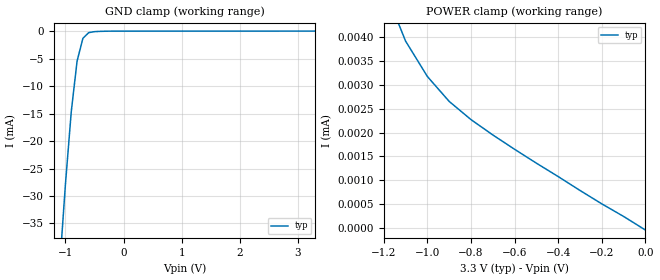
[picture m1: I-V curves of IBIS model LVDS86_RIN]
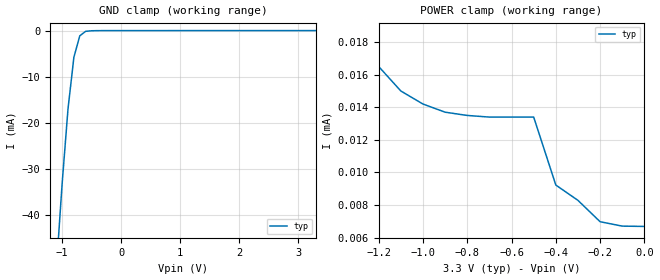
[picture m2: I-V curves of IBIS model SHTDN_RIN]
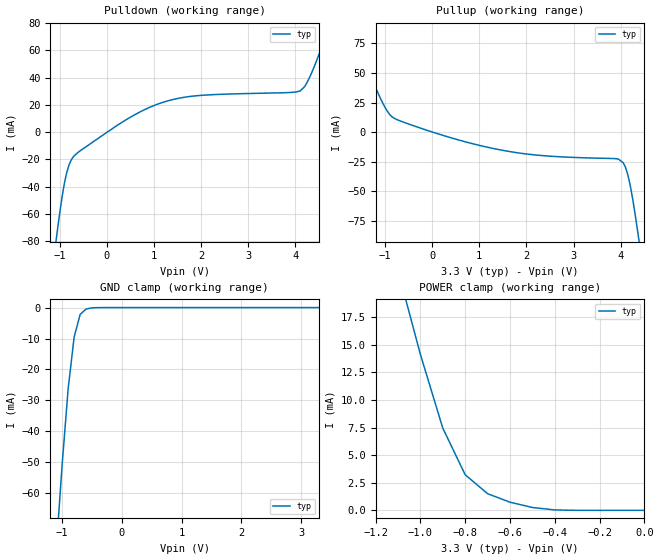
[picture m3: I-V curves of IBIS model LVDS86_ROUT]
|   Texas Instruments Incorporated
|   Data Transmissions Products
|   IBIS Model for SN75LVDS86
|   48DGG Package
[IBIS Ver]   2.1
[Comment char]   |_char
[File name]   75lvds86.ibs
[File Rev]   2.0
[Date]   21Feb97
[Source]   File originated at Texas Instruments Incorporated.
   Data Transmission Products Group. All data based on
   Bench Measurements.
[Notes]   File created by Thomas Fisher
[Disclaimer]
(C) Copyright Texas Instruments Incorporated 1997
   All rights reserved
  Texas Instruments Incorporated hereby grants the user of this IBIS
model a non-exclusive, nontransferable license to use this IBIS model
under the following terms.  Before using this IBIS model, the user
should read this license.  If the user does not accept these terms,
the IBIS model should be returned to Texas Instruments within 30 days.
  The user is granted this license only to use the IBIS model and
is not granted rights to sell, load, rent, lease or license the IBIS
model in whole or in part, or in modified form to anyone other than
user.  User may modify the IBIS model to suit its specific applications
but rights to derivative works and such modifications shall belong to
Texas Instruments.
  This IBIS model is provided on an "AS IS" basis and Texas Instruments
makes absolutely no warranty with respect to the information contained
herein.  TEXAS INSTRUMENTS DISCLAIMS AND CUSTOMER WAIVES ALL WARRANTIES,
EXPRESS OR IMPLIED, INCLUDING WARRANTIES OF MERCHANTABILITY OR FITNESS
FOR A PARTICULAR PURPOSE. The entire risk as to quality and performance
is with the Customer. ACCORDINGLY, IN NO EVENT SHALL THE COMPANY BE LIABLE
FOR ANY DAMAGES, WHETHER IN CONTRACT OR TORT,INCLUDING ANY LOST PROFITS
OR OTHER INCIDENTAL, CONSEQUENTIAL, EXEMPLARY, OR PUNITIVE DAMAGES ARISING
OUT OF THE USE OR APPLICATION OF THE IBIS model provided in this package.
Further, Texas Instruments reserves the right to discontinue or make changes
without notice to any product herein to improve reliability, function, or
design. Texas Instruments does not convey any license under patent rights
or any other intellectual property rights, including those of third parties.
Contact Texas Instruments at ATTN:DATA TRANSMISSIONS
Thomas Fisher  8505 Forest Lane, M/S 8710, Dallas, TX 75243-4136
IBIS Open Forum disclaims all warranties. See DISCLAIM.TXT
in vhdl.org:/pub/IBIS/models for the full disclaimer.
[Copyright]   Copyright 1997, Texas Instruments, All Rights Reserved
[Component]   SN75LVDS86DGG
[Manufacturer]  Texas Instruments Incorporated
[Package]
|   typ   min   max
R_pkg   0.036   0.022   0.041
L_pkg   2.128nH   2.045nH   2.336nH
C_pkg   0.357pF   0.310pF   0.394pF
[Pin]  signal_name   model_name   R_pin   L_pin   C_pin
1   D17   LVDS86_ROUT   0.041   2.221n   0.310p
2   D18   LVDS86_ROUT   0.041   2.297n   0.394p
3   GND   GND   0.022   2.336n   0.380p
4   D19   LVDS86_ROUT   0.031   2.056n   0.343p
5   D20   LVDS86_ROUT   0.034   2.099n   0.383p
6   NC   NC
7   LVDSGND   GND   0.036   2.052n   0.354p
8   A0M   LVDS86_RIN   0.038   2.081n   0.354p
9   A0P   LVDS86_RIN   0.039   2.091n   0.353p
10   A1M   LVDS86_RIN   0.039   2.068n   0.349p
11   A1P   LVDS86_RIN   0.039   2.098n   0.361p
12   LVDSVCC   POWER   0.039   2.100n   0.343p
13   LVDSGND   GND   0.039   2.100n   0.343p
14   A2M   LVDS86_RIN   0.039   2.098n   0.361p
15   A2P   LVDS86_RIN   0.039   2.068n   0.349p
16   CLKINM   LVDS86_RIN   0.039   2.091n   0.353p
17   CLKINP   LVDS86_RIN   0.038   2.081n   0.354p
18   LVDSGND   GND   0.036   2.052n   0.354p
19   PLLGND   GND   0.034   2.045n   0.360p
20   PLLVCC   POWER   0.034   2.099n   0.383p
21   PLLGND   GND   0.031   2.056n   0.343p
22   SHTDN   SHTDN_RIN   0.022   2.330n   0.381p
23   CLKOUT   CLK_OUT   0.041   2.294n   0.394p
24   D0   LVDS86_ROUT   0.041   2.220n   0.310p
25   GND   GND   0.041   2.221n   0.310p
26   D1   LVDS86_ROUT   0.041   2.295n   0.394p
27   D2   LVDS86_ROUT   0.022   2.333n   0.378p
28   VCC   POWER   0.031   2.056n   0.343p
29   D3   LVDS86_ROUT   0.034   2.097n   0.385p
30   D4   LVDS86_ROUT   0.034   2.045n   0.360p
31   D5   LVDS86_ROUT   0.036   2.052n   0.354p
32   GND   GND   0.038   2.080n   0.354p
33   D6   LVDS86_ROUT   0.039   2.090n   0.352p
34   D7   LVDS86_ROUT   0.039   2.067n   0.349p
35   D8   LVDS86_ROUT   0.039   2.097n   0.362p
36   VCC   POWER   0.039   2.100n   0.343p
37   D9   LVDS86_ROUT   0.039   2.100n   0.343p
38   GND   GND   0.039   2.097n   0.362p
39   D10   LVDS86_ROUT   0.039   2.067n   0.349p
40   D11   LVDS86_ROUT   0.039   2.090n   0.352p
41   D12   LVDS86_ROUT   0.038   2.080n   0.354p
42   VCC   POWER   0.036   2.052n   0.354p
43   D13   LVDS86_ROUT   0.034   2.045n   0.360p
44   GND   GND   0.034   2.097n   0.385p
45   D14   LVDS86_ROUT   0.031   2.056n   0.343p
46   D15   LVDS86_ROUT   0.022   2.335n   0.377p
47   D16   LVDS86_RIN   0.041   2.297n   0.394p
48   VCC   POWER   0.041   2.221n   0.310p
[Diff_pin]   inv_pin   vdiff   tdelay_typ   tdelay_min   tdelay_max
| The 'AXP' pin is Diff_pin and the 'AXM' pin is the inv_pin
| The 'CLKINP' pin is Diff_pin and the 'CLKINM' pin is the inv_pin
9   8   100mV   0 0 0   | Vth  +/-100mV
11   10   100mV   0 0 0
15   14   100mV   0 0 0
17   16   100mV   0 0 0
| Models and submodels in the file (4): LVDS86_RIN (Input), SHTDN_RIN (Input), LVDS86_ROUT (3-state), CLK_OUT (3-state)
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|   Receiver Input  MODEL
[Model]   LVDS86_RIN
Model_type   Input
|Signals   A0P,A0M,A1P,A1M,A2P,A2M,CLKINP,CLKINM
Vinh = 2.0
Vinl = 0.8
|   typ   min   max
C_comp   1.8pF   NA   NA
|   typ   min   max
[Temperature Range]   25.0   NA   NA
[Voltage range]   3.3V   3.0V   3.6V
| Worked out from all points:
|   GND clamp passes 1 mA (typ) near -0.67 V on its own axis
[Power_clamp]
| Note that the[POWER_clamp]voltage table is referenced to Vcc
| and is calculated using Vtable=Vcc - Vmeasured.
|   Voltage   I(typ)   I(min)   I(max)
-3.3V     603uA      NA         NA
-1.2V     5.04uA     NA         NA
-1.1V     3.91uA     NA         NA
-1V       3.17uA     NA         NA
-900mV    2.65uA     NA         NA
-800mV    2.27uA     NA         NA
-700mV    1.95uA     NA         NA
-500mV    1.36uA     NA         NA
0V        -36.5nA    NA         NA
[GND_clamp]
|   Voltage   I(typ)   I(min)   I(max)
-3.3V     -401.8mA   NA         NA
-1.1V     -42.95mA   NA         NA
-1V       -27.83mA   NA         NA
-900mV    -14.64mA   NA         NA
-800mV    -5.46mA    NA         NA
-700mV    -1.32mA    NA         NA
-600mV    -280uA     NA         NA
-500mV    -100uA     NA         NA
-200mV    -11.3uA    NA         NA
3.3V      -31.9nA    NA         NA
|   Shutdown/Clear Input  MODEL
[Model]   SHTDN_RIN
Model_type   Input
|Signals   SHTDN
Vinh = 2.0
Vinl = 0.8
|   typ   min   max
C_comp   1.0pF   NA   NA
|   typ   min   max
[Temperature Range]   25.0   NA   NA
[Voltage range]   3.3V   3.0V   3.6V
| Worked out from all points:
|   GND clamp passes 1 mA (typ) near -0.69 V on its own axis
[Power_clamp]
| Note that the[POWER_clamp]voltage table is referenced to Vcc
| and is calculated using Vtable=Vcc - Vmeasured.
|   Voltage   I(typ)   I(min)   I(max)
-3.3V     780uA      NA         NA
-1.3V     19.1uA     NA         NA
-1.2V     16.5uA     NA         NA
-1.1V     15uA       NA         NA
-1V       14.2uA     NA         NA
-900mV    13.7uA     NA         NA
-800mV    13.5uA     NA         NA
-500mV    13.4uA     NA         NA
-400mV    9.23uA     NA         NA
-300mV    8.29uA     NA         NA
-200mV    6.98uA     NA         NA
0V        6.69uA     NA         NA
[GND_clamp]
|   Voltage   I(typ)   I(min)   I(max)
-3.3V     -485.8mA   NA         NA
-1.1V     -52.3mA    NA         NA
-1V       -33.38mA   NA         NA
-900mV    -17.03mA   NA         NA
-800mV    -5.78mA    NA         NA
-700mV    -1.13mA    NA         NA
-600mV    -150uA     NA         NA
-300mV    -2.96uA    NA         NA
3.3V      6.69uA     NA         NA
|   Receiver Output  MODEL
[Model]   LVDS86_ROUT
Model_type   3-state
| Signals   D0,D1,D2,D3,D4,D5,D6,D7,D8,D9,D10,D11,D12,D13,D14,D15,D16,D17
|   D18,D19,D20
Vmeas = 1.5V   |Reference voltage for timing measurements
Cref = 8pF   |Timing specification test load capacitance value
Vref = 0   |Timing specification test load voltage; GND
| variable   typ   min   max
C_comp   1.2pF   NA   NA
|   typ   min   max
[Temperature Range]   25.0   NA   NA
[Voltage range]   3.3V   3.0V   3.6V
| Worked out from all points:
|   slope of the pulldown table from 0 to 0.495 V, typ, clamps not added: 44.9 ohm
|   slope of the pullup table from 0 to 0.495 V, typ, clamps not added: 82.4 ohm
|   GND clamp passes 1 mA (typ) near -0.63 V on its own axis
|   POWER clamp passes 1 mA (typ) near -0.63 V on its own axis
[Pulldown]
|   Voltage   I(typ)   I(min)   I(max)
-3.3V     -585.2mA   NA         NA
-1.1V     -85.54mA   NA         NA
-1.05V    -72.24mA   NA         NA
-900mV    -37.39mA   NA         NA
-750mV    -20.06mA   NA         NA
500mV     10.93mA    NA         NA
1.1V      20.79mA    NA         NA
1.7V      25.83mA    NA         NA
4.1V      30.15mA    NA         NA
4.3V      40.15mA    NA         NA
4.6V      66.91mA    NA         NA
6.6V      266.1mA    NA         NA
[Pullup]
|   Voltage   I(typ)   I(min)   I(max)
| Note that the[Pullup]voltage table is referenced to Vcc
| and is calculated using Vtable=Vcc - Vmeasured.
-3.3V     231.2mA    NA         NA
-1.2V     37.7mA     NA         NA
-900mV    14.78mA    NA         NA
-700mV    9.785mA    NA         NA
1.55V     -15.8mA    NA         NA
3.95V     -22.85mA   NA         NA
4.05V     -25.83mA   NA         NA
4.15V     -36.24mA   NA         NA
4.25V     -56.07mA   NA         NA
4.35V     -81.84mA   NA         NA
4.4V      -95.55mA   NA         NA
6.6V      -698.8mA   NA         NA
[GND_clamp]
|   Voltage   I(typ)   I(min)   I(max)
| Outputs in Tri-state.
-3.3V     -689.8mA   NA         NA
-1.1V     -78.22mA   NA         NA
-1V       -50.42mA   NA         NA
-900mV    -26.09mA   NA         NA
-800mV    -9.48mA    NA         NA
-700mV    -2.23mA    NA         NA
-600mV    -460uA     NA         NA
-500mV    -91.7uA    NA         NA
-300mV    -2.58uA    NA         NA
3.3V      900pA      NA         NA
[POWER_clamp]
|   Voltage   I(typ)   I(min)   I(max)
| Note that the [POWER_clamp] voltage table is referenced to Vcc
| and is calculated using Vtable = Vcc - Vmeasured.
| Outputs in Tri-state.
-3.3V     208.5mA    NA         NA
-1.1V     21.72mA    NA         NA
-1V       14.13mA    NA         NA
-900mV    7.445mA    NA         NA
-800mV    3.224mA    NA         NA
-700mV    1.51mA     NA         NA
-600mV    739uA      NA         NA
-500mV    260uA      NA         NA
-400mV    38.9uA     NA         NA
0V        -9.18nA    NA         NA
[Ramp]
|   typ   min   max
dV/dt_r   1.876v/1115ps   NA   NA
dV/dt_f   1.905v/1200ps   NA   NA
R_load = 1000ohm
